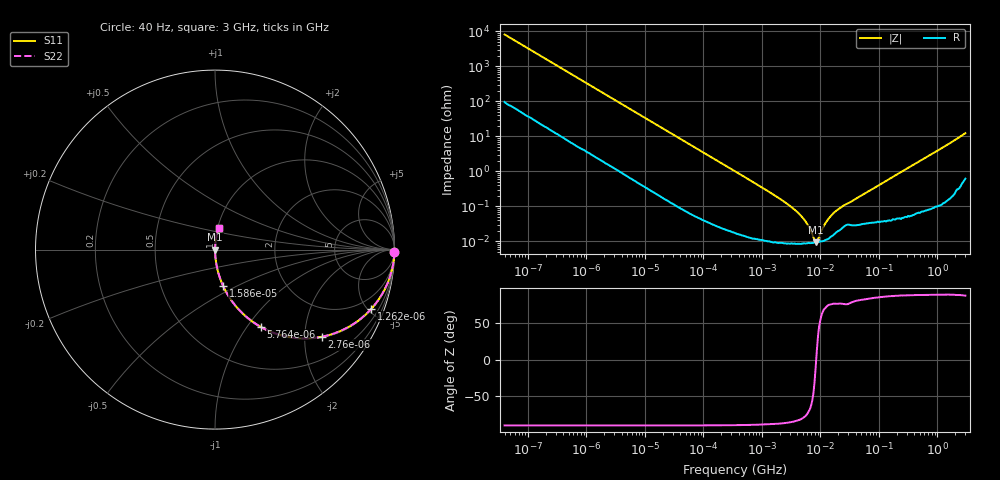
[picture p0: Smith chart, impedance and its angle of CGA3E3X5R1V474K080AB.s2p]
! S-parameter Generated by TDK Corporation
! Copyright(C) 2015 TDK Corporation.
! All Rights Reserved.
! TDK P/N: CGA3E3X5R1V474K080AB (Multilayer Ceramic Chip Capacitors)
! Property: C=470nF
! Size(LxWxT): 1.6x0.8x0.8mm, 0.063x0.031x0.031inches
! Model Type: s2p (Touchstone File Format Version 1.0)
! Frequency: DC=Yes Start=0.00004MHz Stop=3000MHz 396points Log-sweep
! Note: This model was converted from impedance.
! Model Generated on Jun. 23, 2015
! Hash(MD5):
! Port Assignments:
!  1 ---| |--- 2
! Applicable Conditions:
!  Temperature = 25 degC
!  DC Bias Voltage = 0 V
!  Small Signal Operation
! Terms and conditions regarding TDK Simulation Models
! (1)This simulation model is being provided solely for informational purposes. Please refer to the specifications of the products in terms of detailed characteristics of such products.
! (2)In no event shall TDK Corporation of any of its subsidiaries be liable for any loss or damage arising, directly or indirectly,
!  From any information contained in this simulation model, including, but not limited to loss or damages arising from any inaccuracies, omissions or errors in connection with such information.
! (3)Any and all copyrights on this simulation model are owned by TDK Corporation.
!  Duplication or redistribution of this simulation model without prior written permission from TDK Corporation is prohibited.
! (4)This simulation model is subject to any modification or change without any prior notice.
! (5)Neither TDK Corporation nor any of its subsidiaries shall make any warranty, express or implied,
!  Including but not limited to the correctness, implied warranties of merchantability and fitness for a particular purpose with respect to this simulation models.
! (6)The use of this simulation model shall be deemed to have consented to the terms and conditions hereof.
# MHz S MA R 50
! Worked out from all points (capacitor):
!   395 points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, 40 Hz to 3 GHz, reference 50 ohm
!   read as one part in series: C = 488 nF near 41.88 Hz
!   lowest |Z| = 9.42 mohm at 8.293 MHz (marker M1)
!   series resonance near 8.46 MHz, so ESL is about 730 pH
!   S11 on the Smith chart (normalised r, x): 40 Hz: open; 1.262 kHz: 1.06, -5.28; 2.76 kHz: 1.03, -2.43; 5.764 kHz: 1.01, -1.17; 15.86 kHz: 1.00, -0.43; 3 GHz: 1.01, +0.25
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4e-05  0.9998 -0.7  0.01227 88.6  0.01227 88.6  0.9998 -0.7
0.0002520917  0.9962 -4.4  0.07618 85.0  0.07618 85.0  0.9962 -4.4
0.000834128  0.9674 -14.1  0.243 75.3  0.243 75.3  0.9674 -14.1
0.001262176  0.9317 -20.7  0.3531 68.7  0.3531 68.7  0.9317 -20.7
0.002759985  0.7676 -39.2  0.6327 50.1  0.6327 50.1  0.7676 -39.2
0.005763764  0.5021 -59.3  0.8595 30.1  0.8595 30.1  0.5021 -59.3
0.009132315  0.3461 -69.2  0.9346 20.2  0.9346 20.2  0.3461 -69.2
0.01586465  0.2091 -77.3  0.9757 12.1  0.9757 12.1  0.2091 -77.3
0.01739424  0.1916 -78.4  0.9795 11.0  0.9795 11.0  0.1916 -78.4
0.05755453  0.05976 -86.0  0.9976 3.4  0.9976 3.4  0.05976 -86.0
0.3464102  0.01008 -88.4  0.9998 0.6  0.9998 0.6  0.01008 -88.4
3.459106  0.0008573 -84.2  0.9999 0.0  0.9999 0.0  0.0008573 -84.2
5.480732  0.000386 -77.0  0.9999 0.0  0.9999 0.0  0.000386 -77.0
7.22376  0.000162 -56.0  0.9999 0.0  0.9999 0.0  0.000162 -56.0
8.293268  9.415e-05 -10.0  0.9999 0.0  0.9999 0.0  9.415e-05 -10.0
9.092863  0.0001148 32.4  0.9999 -0.0  0.9999 -0.0  0.0001148 32.4
10.4391  0.0002048 60.7  0.9999 -0.0  0.9999 -0.0  0.0002048 60.7
12.54911  0.0003565 71.6  0.9999 -0.0  0.9999 -0.0  0.0003565 71.6
18.13479  0.0007238 76.1  0.9998 -0.0  0.9998 -0.0  0.0007238 76.1
150.6385  0.006094 85.9  0.9996 -0.3  0.9996 -0.3  0.006094 85.9
994.0817  0.03878 86.3  0.9982 -2.2  0.9982 -2.2  0.03878 86.3
3000  0.1221 80.1  0.9864 -7.0  0.9864 -7.0  0.1221 80.1
